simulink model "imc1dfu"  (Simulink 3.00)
settings: Solver=ode45  SolverMode=SingleTasking  StartTime=0.0  StopTime=50  MaxStep=st_size  RelTol=1e-5  AbsTol=1e-6
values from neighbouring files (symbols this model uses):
  Disturb = Setpoint    [mimo_MSF1DF_sim.m]    (also in mimo_MSF2DF_sim.m)
  Satlb = temp1    [cback.m]    (also in imcmenu.m = str2num(satlbs))
  Satub = temp1    [cback.m]    (also in imcmenu.m = str2num(satubs))
  Setpoint = zeros(1,n)    [mimo_MSF1DF_sim.m]    (also in mimo_MSF2DF_sim.m)
undefined symbols (not defined in the file or in its folder): Csden, Csnum, denPs, numPs, Pdelay

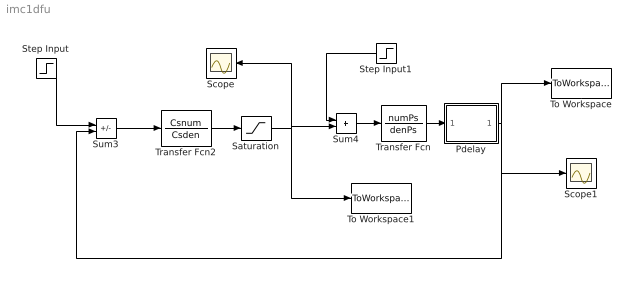
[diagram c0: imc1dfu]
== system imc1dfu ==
  Pdelay : Subsystem
  Saturation : Saturate  UpperLimit=Satub  LowerLimit=Satlb
  Scope : Scope
  Scope1 : Scope
  Step Input : Step  Time=0  Before=0  After=Setpoint  SampleTime=0
  Step Input1 : Step  Orientation=left  Time=0  Before=0  After=Disturb  SampleTime=0
  Sum3 : Sum  Inputs=+-  SaturateOnIntegerOverflow=on
  Sum4 : Sum  Inputs=++  SaturateOnIntegerOverflow=on
  To Workspace : ToWorkspace  VariableName=simout  SampleTime=-1  SaveFormat=Matrix
  To Workspace1 : ToWorkspace  VariableName=effort  SampleTime=-1  SaveFormat=Matrix
  Transfer Fcn : TransferFcn  Numerator=numPs  Denominator=denPs
  Transfer Fcn2 : TransferFcn  Numerator=Csnum  Denominator=Csden
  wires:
  Sum3/1 -> Transfer Fcn2/1
  Transfer Fcn/1 -> Pdelay/1(In1)
  Transfer Fcn2/1 -> Saturation/1
  Step Input/1 -> Sum3/1
  Step Input1/1 -> Sum4/1
  Sum4/1 -> Transfer Fcn/1
  Saturation/1 -> Sum4/2, Scope/1, To Workspace1/1
  Pdelay/1(Out1) -> Sum3/2, To Workspace/1, Scope1/1

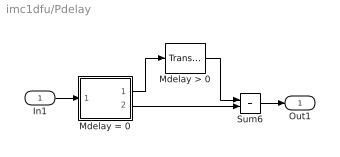
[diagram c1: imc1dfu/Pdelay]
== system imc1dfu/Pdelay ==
  In1 : Inport  Port=1  PortWidth=-1  SampleTime=-1  DataType=auto
  Mdelay > 0 : TransportDelay  DelayTime=Pdelay  InitialInput=0  BufferSize=1024
  Mdelay = 0 : Subsystem  Description=pass input signal through out1 if condition is true.
  Sum6 : Sum  Inputs=++  SaturateOnIntegerOverflow=on
  Out1 : Outport  Port=1
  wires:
  Mdelay = 0/1(Out2) -> Mdelay > 0/1
  Mdelay > 0/1 -> Sum6/1
  Mdelay = 0/2(Out1) -> Sum6/2
  In1/1 -> Mdelay = 0/1(In)
  Sum6/1 -> Out1/1

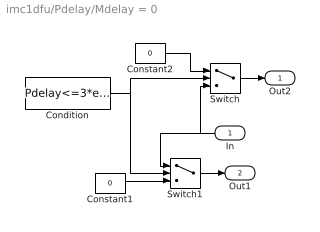
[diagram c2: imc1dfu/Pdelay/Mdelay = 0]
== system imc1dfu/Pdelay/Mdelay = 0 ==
  In : Inport  Orientation=left  Port=1  PortWidth=-1  SampleTime=-1  DataType=auto
  Condition : Constant  Value=Pdelay<=3*eps
  Constant1 : Constant  Value=0
  Constant2 : Constant  Value=0
  Switch : Switch  Threshold=1
  Switch1 : Switch  Threshold=1
  Out2 : Outport  Port=1  InitialOutput=0
  Out1 : Outport  Port=2  InitialOutput=0
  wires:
  In/1 -> Switch/3, Switch1/1
  Condition/1 -> Switch1/2, Switch/2
  Constant1/1 -> Switch1/3
  Constant2/1 -> Switch/1
  Switch/1 -> Out2/1
  Switch1/1 -> Out1/1
